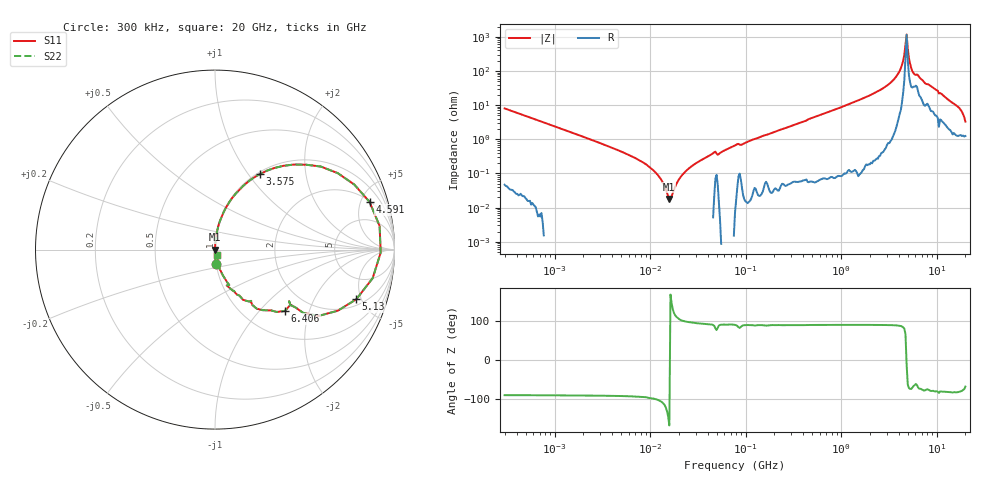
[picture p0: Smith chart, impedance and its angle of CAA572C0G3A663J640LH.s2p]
! S-Parameter Data Generated by TDK Corporation
! Copyright(C) 2022 TDK Corporation.
! All Rights Reserved.
! TDK P/N: CAA572C0G3A663J640LH (Multilayer Ceramic Chip Capacitor)
! Property: C=66nF
! Size(LxWxT): 6x5.6x6.4mm
! Model Type: s2p (Touchstone File Format Version 1.0)
! Frequency: DC=Yes Start=0.3MHz Stop=20000MHz 402points Log-sweep
! Model Generated on Apr. 15, 2022
! Port Assignments:
!  1 ---| |--- 2
! Applicable Conditions:
!  Temperature = 25 degC
!  DC Bias Voltage = 0 V
!  Small Signal Operation
! Terms and conditions regarding TDK Simulation Models
! (1)This simulation model is being provided solely for informational purposes. Please refer to the specifications of the products in terms of detailed characteristics of such products.
! (2)In no event shall TDK Corporation of any of its subsidiaries be liable for any loss or damage arising, directly or indirectly,
!  From any information contained in this simulation model, including, but not limited to loss or damages arising from any inaccuracies, omissions or errors in connection with such information.
! (3)Any and all copyrights on this simulation model are owned by TDK Corporation.
!  Duplication or redistribution of this simulation model without prior written permission from TDK Corporation is prohibited.
! (4)This simulation model is subject to any modification or change without any prior notice.
! (5)Neither TDK Corporation nor any of its subsidiaries shall make any warranty, express or implied,
!  Including but not limited to the correctness, implied warranties of merchantability and fitness for a particular purpose with respect to this simulation models.
! (6)The use of this simulation model shall be deemed to have consented to the terms and conditions hereof.
# Hz S MA R 50
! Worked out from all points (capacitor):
!   401 points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, 300 kHz to 20 GHz, reference 50 ohm
!   read as one part in series: C = 66 nF near 317.1 kHz
!   lowest |Z| = 18 mohm at 15.91 MHz (marker M1)
!   series resonance near 16.13 MHz, so ESL is about 1.5 nH
!   S11 on the Smith chart (normalised r, x): 300 kHz: 1.00, -0.16; 3.575 GHz: 1.03, +1.14; 4.591 GHz: 2.09, +5.91; 5.13 GHz: 2.49, -4.53; 6.406 GHz: 1.49, -1.40; 20 GHz: 1.03, -0.06
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300000  0.08007 -85.1  0.9963 4.6  0.9963 4.6  0.08007 -85.1
1928084  0.01231 -89.9  1 0.7  1 0.7  0.01231 -89.9
7111075  0.00276 -93.2  1 0.2  1 0.2  0.00276 -93.2
1.239169e7  0.0008179 -103.0  1 0.0  1 0.0  0.0008179 -103.0
1.590994e7  0.0001804 -166.9  1 0.0  1 0.0  0.0001804 -166.9
2.100228e7  0.000806 101.5  1 -0.0  1 -0.0  0.000806 101.5
2.622675e7  0.001502 96.0  1 -0.1  1 -0.1  0.001502 96.0
4.57025e7  0.003915 89.0  0.9999 -0.2  0.9999 -0.2  0.003915 89.0
7.964076e7  0.006921 88.2  0.9998 -0.4  0.9998 -0.4  0.006921 88.2
4.978292e8  0.04247 86.8  0.9985 -2.4  0.9985 -2.4  0.04247 86.8
1.643049e9  0.1509 80.9  0.9875 -8.7  0.9875 -8.7  0.1509 80.9
3.199522e9  0.3878 66.1  0.9146 -22.8  0.9146 -22.8  0.3878 66.1
3.575396e9  0.4902 59.2  0.8592 -29.3  0.8592 -29.3  0.4902 59.2
4.2236e9  0.7497 38.1  0.6182 -48.4  0.6182 -48.4  0.7497 38.1
4.590522e9  0.9013 17.2  0.2999 -62.4  0.2999 -62.4  0.9013 17.2
4.85268e9  0.9234 -1.0  0.07848 12.0  0.07848 12.0  0.9234 -1.0
5.129809e9  0.8342 -19.4  0.3496 52.4  0.3496 52.4  0.8342 -19.4
5.575457e9  0.6037 -35.7  0.6194 34.6  0.6194 34.6  0.6037 -35.7
6.405888e9  0.5181 -41.3  0.6998 29.2  0.6998 29.2  0.5181 -41.3
9.989315e9  0.2536 -65.3  0.9232 14.4  0.9232 14.4  0.2536 -65.3
1.646689e10  0.09156 -77.0  0.9835 5.2  0.9835 5.2  0.09156 -77.0
2e10  0.03265 -66.1  0.9872 1.7  0.9872 1.7  0.03265 -66.1
